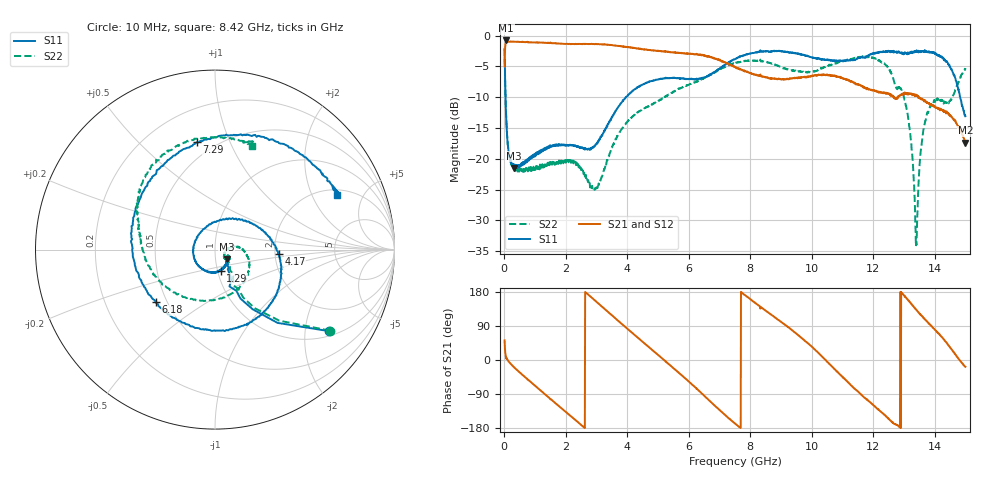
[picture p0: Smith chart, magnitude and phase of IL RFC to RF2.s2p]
!Agilent Technologies,N5230A,MY45001650,A.07.50.48
!Agilent N5230A: A.07.50.48
!Date: Wednesday, April 30, 2014 16:47:00
!Correction: S11(Full 2 Port(1,2))
!S21(Full 2 Port(1,2))
!S12(Full 2 Port(1,2))
!S22(Full 2 Port(1,2))
!S2P File: Measurements: S11, S21, S12, S22:
# Hz S  dB  R 50
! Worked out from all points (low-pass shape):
!   1500 points, 10 MHz to 15 GHz, reference 50 ohm
!   highest |S21| = -0.79 dB at 60 MHz (marker M1); lowest = -17.4 dB at 15 GHz (marker M2)
!   |S21| within 3 dB of the highest: 15.33 MHz to 6.896 GHz (6.88 GHz wide, 199 % of centre)
!   lowest |S11| = -21.5 dB at 300 MHz (marker M3), VSWR 1.18, Z = 56.6 - j6.15 ohm
!   |S11| at or under -10 dB: 38.92 MHz to 3.962 GHz (3.923 GHz wide, 196 % of centre); 14.83 GHz to end of sweep
!   |S22| runs from -34.2 to -2.1 dB; largest |S21 - S12| = 0.011
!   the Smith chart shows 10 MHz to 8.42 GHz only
!   S11 on the Smith chart (normalised r, x): 10 MHz: 1.15, -2.68; 1.29 GHz: 1.04, -0.25; 4.17 GHz: 2.10, -0.12; 6.18 GHz: 0.43, -0.32; 7.29 GHz: 0.40, +0.76; 8.42 GHz: 2.30, +3.13
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1e7  -2.15 -35.6  -4.99 51.8  -5.01 51.8  -2.12 -35.2
6e7  -13.13 -68.6  -0.79 3.9  -0.81 3.9  -12.98 -62.7
3e8  -21.49 -39.8  -0.97 -17.9  -0.99 -17.8  -21.33 -30.7
1.29e9  -18.33 -74.6  -1.17 -88.0  -1.16 -88.1  -20.92 -28.5
2.51e9  -18.15 -170.9  -1.37 -172.0  -1.35 -172.0  -21.81 -42.5
3.44e9  -13.83 57.0  -1.50 122.3  -1.53 122.4  -19.03 7.8
4.17e9  -8.96 -3.9  -1.95 70.9  -1.96 70.9  -13.17 -30.7
5.01e9  -7.10 -52.2  -2.52 12.9  -2.49 12.9  -10.58 -106.1
6.18e9  -7.10 -138.3  -3.04 -69.8  -3.05 -69.9  -7.64 173.3
7.29e9  -4.34 99.6  -4.58 -152.9  -4.57 -153.0  -4.80 130.7
7.51e9  -3.82 81.4  -5.11 -168.0  -5.18 -167.8  -4.46 120.1
8.42e9  -2.55 24.0  -6.67 135.3  -6.73 135.3  -4.21 70.2
1.001e10  -3.53 -65.9  -6.52 34.6  -6.55 34.6  -5.90 -45.5
1.061e10  -4.01 -115.2  -6.44 -12.8  -6.44 -12.6  -4.83 -85.8
1.122e10  -4.02 179.1  -7.36 -61.8  -7.31 -62.0  -3.92 -117.1
1.194e10  -2.95 111.9  -8.79 -114.2  -8.69 -114.4  -3.60 -147.5
1.251e10  -2.56 73.3  -9.38 -155.7  -9.42 -155.6  -5.24 -173.6
1.309e10  -2.87 48.3  -9.39 162.2  -9.48 162.9  -12.02 160.7
1.34e10  -2.64 39.8  -9.71 132.9  -9.82 133.3  -33.78 49.3
1.378e10  -2.57 24.7  -10.97 98.7  -10.82 99.2  -12.47 -52.6
1.441e10  -4.33 -9.2  -12.61 43.7  -12.58 43.6  -11.09 -51.5
1.5e10  -13.09 -121.3  -17.41 -17.9  -17.37 -18.5  -5.27 -28.6
